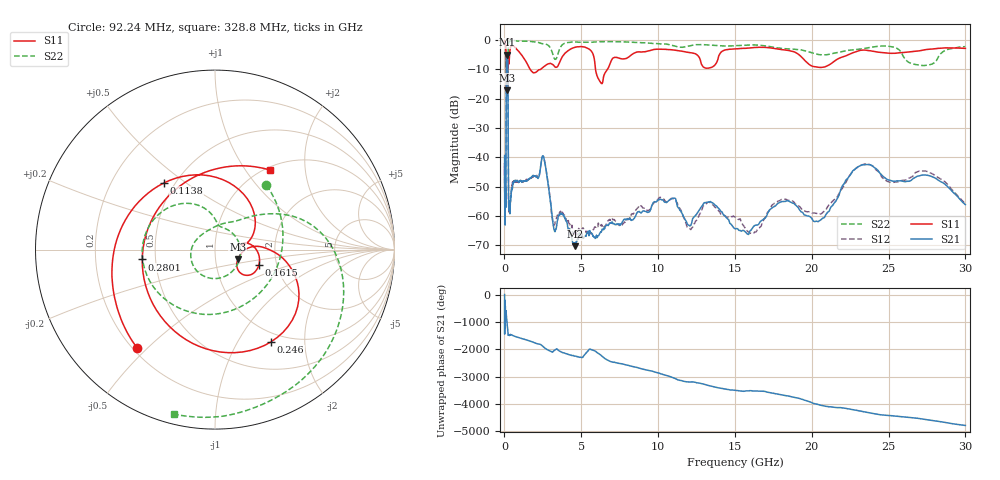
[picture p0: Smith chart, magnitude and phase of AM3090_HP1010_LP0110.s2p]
! Date/Time: Thu, Feb 28, 2019 2:04 PM
! Network Analyzer: Agilent Technologies E8364B Rev: A.07.50.67
! Sweep from 0.010 to 30.000 GHz, 1601 Points, Sweep Type: LOG
! Power Supply: 5.022 V, 0.002 A
# Hz S DB R 50
!freq MagS11 AngS11 MagS21 AngS21 MagS12 AngS12 MagS22 AngS22
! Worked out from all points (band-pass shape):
!   1601 points, 10 MHz to 30 GHz, reference 50 ohm
!   highest |S21| = -5.05 dB at 165.6 MHz (marker M1); lowest = -70.3 dB at 4.617 GHz (marker M2)
!   |S21| within 3 dB of the highest: 127.5 MHz to 214 MHz (86.43 MHz wide, 50.6 % of centre)
!   lowest |S11| = -17.2 dB at 197.3 MHz (marker M3), VSWR 1.32, Z = 64.1 - j7.06 ohm
!   |S11| at or under -10 dB: 123 MHz to 220.1 MHz (97.09 MHz wide, 56.6 % of centre); 1.669 GHz to 2.364 GHz (694.9 MHz wide, 34.5 % of centre); 5.927 GHz to 6.71 GHz (782.8 MHz wide, 12.4 % of centre)
!   |S22| runs from -19.1 to -0.2 dB; largest |S21 - S12| = 0.016
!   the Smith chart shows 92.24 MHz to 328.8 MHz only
!   S11 on the Smith chart (normalised r, x): 92.24 MHz: 0.22, -0.47; 113.8 MHz: 0.44, +0.41; 161.5 MHz: 1.61, -0.30; 246 MHz: 0.87, -1.40; 280.1 MHz: 0.42, -0.06; 328.8 MHz: 1.05, +1.31
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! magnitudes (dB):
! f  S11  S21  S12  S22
! 10 MHz  -0.2  -39.4  -44.0  -0.5
! 38.04 MHz  -0.5  -58.0  -60.2  -1.4
! 92.24 MHz  -3.1  -53.8  -54.0  -6.8
! 113.8 MHz  -6.6  -19.9  -19.9  -7.9
! 144.7 MHz  -14.1  -5.5  -5.4  -17.6
! 161.5 MHz  -11.7  -5.1  -5.0  -16.3
! 165.6 MHz  -11.8  -5.1  -5.0  -16.0
! 197.3 MHz  -17.2  -5.9  -5.9  -19.1
! 223.6 MHz  -9.0  -11.8  -11.8  -11.6
! 246 MHz  -4.4  -37.7  -37.7  -2.8
! 280.1 MHz  -7.8  -56.9  -57.3  -1.0
! 328.8 MHz  -5.4  -56.1  -58.5  -0.5
! 550.5 MHz  -2.0  -49.1  -48.6  -0.3
! 2.084 GHz  -10.9  -46.6  -46.3  -0.7
! 2.545 GHz  -9.2  -39.8  -39.9  -1.3
! 3.236 GHz  -8.9  -64.7  -63.1  -6.3
! 4.617 GHz  -2.5  -70.3  -65.9  -0.7
! 7.926 GHz  -6.3  -61.2  -62.0  -0.7
! 16.13 GHz  -2.7  -64.2  -66.0  -1.7
! 20.61 GHz  -9.4  -61.3  -59.3  -5.1
! 23.48 GHz  -3.5  -42.6  -42.3  -2.9
! 30 GHz  -2.9  -56.2  -55.9  -2.3
